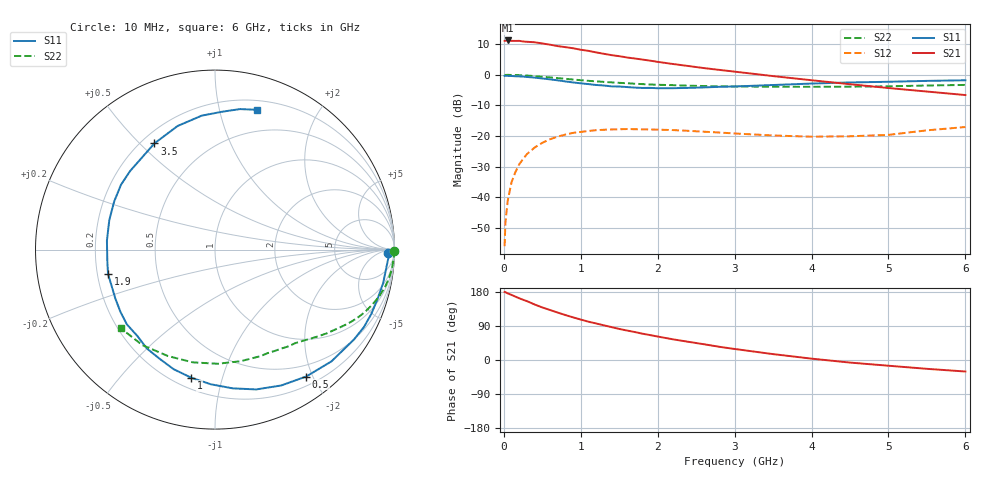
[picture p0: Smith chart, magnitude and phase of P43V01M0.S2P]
! SIEMENS Small Signal Semiconductors
! BFP182
! Si NPN RF Bipolar Junction Transistor in SOT143
! VCE = 3 V  IC = 1 mA
! Common Emitter S-Parameters:  March  1996
# GHz  S  MA  R  50
!  f  S11  S21  S12  S22
! GHz  MAG  ANG  MAG  ANG  MAG  ANG  MAG  ANG
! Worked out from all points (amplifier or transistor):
!   36 points, 10 MHz to 6 GHz, reference 50 ohm
!   highest |S21| = 11.2 dB at 50 MHz (marker M1)
!   |S21| within 3 dB of that: start of sweep to 994.9 MHz
!   unconditionally stable (mu >= 1): 2.633 GHz to end of sweep
!   at 250 MHz: K = 0.10, MSG = 19.2 dB, |S12| = -27.5 dB
!   at 1.4 GHz: K = 0.54, MSG = 12.1 dB, |S12| = -17.8 dB
!   at 6 GHz: K = 1.06, MAG = 3.7 dB, |S12| = -17.0 dB
!   S11 on the Smith chart (normalised r, x): 10 MHz: 43, -20; 500 MHz: 0.33, -1.91; 1 GHz: 0.26, -0.80; 1.9 GHz: 0.24, -0.11; 3.5 GHz: 0.25, +0.55; 6 GHz: 0.28, +1.31
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0.01  0.9622 -1.0  3.579 179.5  0.0016 80.8  0.9984 -0.4
0.02  0.9684 -2.3  3.589 179.0  0.0038 89.4  0.9937 -0.8
0.05  0.9604 -5.7  3.632 175.8  0.0088 89.5  0.9982 -2.0
0.1  0.9554 -11.2  3.58 171.7  0.0177 81.9  0.9939 -4.2
0.2  0.9419 -22.4  3.576 162.9  0.0347 75.9  0.9855 -8.2
0.4  0.8993 -43.8  3.394 146.5  0.065 63.2  0.9521 -15.8
0.5  0.8707 -54.3  3.246 138.7  0.0776 57.0  0.9285 -19.3
0.6  0.8422 -64.0  3.098 132.0  0.0888 51.3  0.9062 -22.4
0.8  0.7794 -82.7  2.825 118.6  0.1058 41.2  0.8597 -27.8
0.9  0.7506 -91.8  2.71 112.5  0.1128 36.7  0.8374 -30.1
1  0.726 -100.5  2.564 106.7  0.1168 32.6  0.8158 -32.4
1.1  0.705 -109.1  2.458 101.1  0.1213 28.8  0.7974 -34.4
1.3  0.6691 -124.6  2.2 91.5  0.1268 22.1  0.7658 -38.2
1.5  0.6439 -139.7  2.012 82.0  0.1293 16.7  0.7391 -41.4
1.9  0.6114 -167.1  1.701 65.8  0.1282 7.9  0.6954 -47.9
2.2  0.6042 175.3  1.499 54.5  0.1253 3.2  0.6776 -52.6
2.8  0.6363 145.4  1.203 34.9  0.1144 -2.2  0.6474 -62.9
3.5  0.6812 119.7  0.952 15.5  0.1023 -2.3  0.638 -77.1
4  0.7196 106.8  0.815 3.6  0.0978 2.1  0.6362 -88.7
4.5  0.7499 95.7  0.702 -6.8  0.0993 7.3  0.6403 -101.2
5.5  0.7952 79.9  0.533 -23.3  0.1241 16.3  0.6686 -127.3
6  0.8139 73.1  0.467 -30.4  0.1406 15.1  0.6835 -140.1
